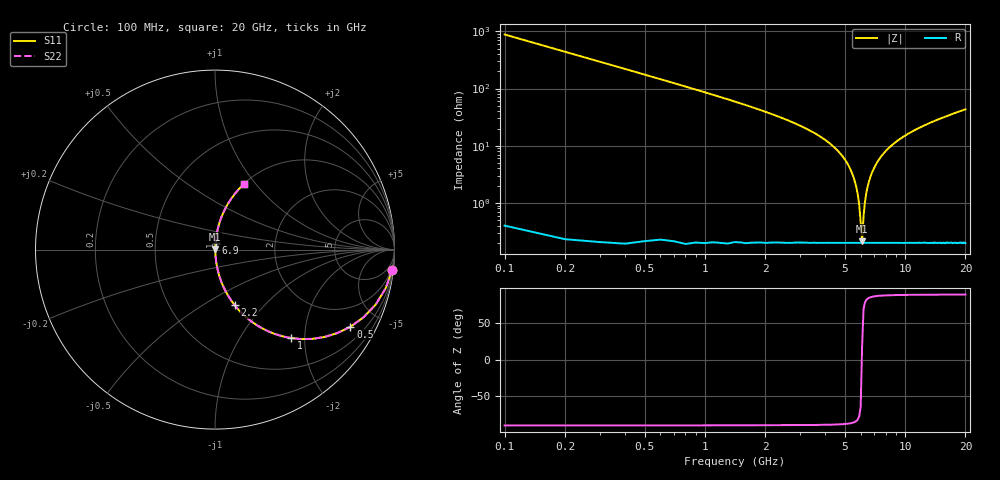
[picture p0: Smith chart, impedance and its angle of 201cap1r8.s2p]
! AVX Thin Film Operation		Date: May 2007
! Description: Accu-P® Series, Thin Film, SMD, RF Capacitor
! Part Number: 02013J1R8ABS
! 50 MHz  -  20.05 GHz
! Serial Measurements
# hz S db R 50
!	S11		S21		S12		S22
!	dB	Phase	dB	Phase	dB	Phase	dB	Phase
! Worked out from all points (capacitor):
!   200 points, 100 MHz to 20 GHz, reference 50 ohm
!   read as one part in series: C = 1.8 pF near 200 MHz
!   lowest |Z| = 212 mohm at 6.1 GHz (marker M1)
!   series resonance near 6.086 GHz, so ESL is about 380 pH
!   S11 on the Smith chart (normalised r, x): 100 MHz: 1, -18; 500 MHz: 1.00, -3.51; 1 GHz: 1.00, -1.72; 2.2 GHz: 1.00, -0.70; 6.9 GHz: 1.00, +0.07; 20 GHz: 1.00, +0.87
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1e8  -0.06 -6.5  -18.98 83.5  -18.98 83.5  -0.06 -6.5
2e8  -0.22 -12.8  -13.12 77.2  -13.12 77.2  -0.22 -12.8
3e8  -0.48 -18.8  -9.85 71.2  -9.85 71.2  -0.48 -18.8
5e8  -1.22 -29.6  -6.12 60.3  -6.12 60.3  -1.22 -29.6
1e9  -3.72 -49.2  -2.42 40.6  -2.42 40.6  -3.72 -49.2
2.2e9  -9.65 -70.5  -0.52 19.2  -0.52 19.2  -9.65 -70.5
3.5e9  -15.58 -79.7  -0.14 9.6  -0.14 9.6  -15.58 -79.7
4.8e9  -23.18 -84.4  -0.04 4.0  -0.04 4.0  -23.18 -84.4
5.5e9  -30.62 -84.4  -0.02 1.7  -0.02 1.7  -30.62 -84.4
5.7e9  -34.38 -82.9  -0.02 1.1  -0.02 1.1  -34.38 -82.9
5.9e9  -40.73 -77.0  -0.02 0.5  -0.02 0.5  -40.73 -77.0
6.1e9  -53.50 19.1  -0.02 -0.0  -0.02 -0.0  -53.50 19.1
6.2e9  -44.78 69.4  -0.02 -0.3  -0.02 -0.3  -44.78 69.4
6.3e9  -39.79 78.2  -0.02 -0.6  -0.02 -0.6  -39.79 78.2
6.5e9  -34.32 83.0  -0.02 -1.1  -0.02 -1.1  -34.32 83.0
6.8e9  -29.81 84.6  -0.02 -1.8  -0.02 -1.8  -29.81 84.6
6.9e9  -28.74 84.8  -0.02 -2.1  -0.02 -2.1  -28.74 84.8
8.1e9  -21.54 83.8  -0.05 -4.8  -0.05 -4.8  -21.54 83.8
1.01e10  -16.39 80.5  -0.12 -8.7  -0.12 -8.7  -16.39 80.5
1.34e10  -12.19 75.3  -0.29 -14.2  -0.29 -14.2  -12.19 75.3
1.67e10  -9.73 70.6  -0.51 -19.0  -0.51 -19.0  -9.73 70.6
2e10  -8.03 66.3  -0.76 -23.4  -0.76 -23.4  -8.03 66.3
